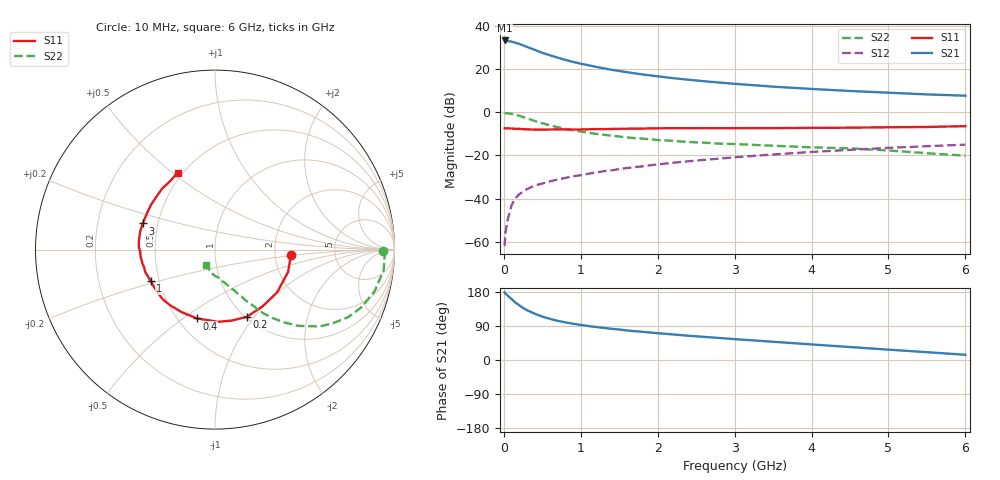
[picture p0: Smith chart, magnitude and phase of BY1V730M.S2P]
! SIEMENS Small Signal Semiconductors
! BFY420
! Si NPN RF SIEGET Grounded Emitter Transistor in MICRO-X
! VCE = 1.75 V  IC = 30 mA
! Common Emitter S-Parameters:  October  1996
# GHz  S  MA  R  50
!  f  S11  S21  S12  S22
! GHz  MAG  ANG  MAG  ANG  MAG  ANG  MAG  ANG
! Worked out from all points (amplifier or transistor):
!   36 points, 10 MHz to 6 GHz, reference 50 ohm
!   highest |S21| = 33.2 dB at 10 MHz (marker M1)
!   |S21| within 3 dB of that: start of sweep to 302.7 MHz
!   unconditionally stable (mu >= 1): start of sweep to 12.17 MHz; 1.57 GHz to end of sweep
!   at 250 MHz: K = 0.37, MSG = 33.8 dB, |S12| = -36.8 dB
!   at 1.4 GHz: K = 0.98, MSG = 23.3 dB, |S12| = -26.9 dB
!   at 6 GHz: K = 1.07, MAG = 9.7 dB, |S12| = -15.0 dB
!   S11 on the Smith chart (normalised r, x): 10 MHz: 2.47, -0.19; 200 MHz: 1.02, -0.92; 400 MHz: 0.62, -0.56; 1 GHz: 0.45, -0.19; 3 GHz: 0.41, +0.15; 6 GHz: 0.47, +0.52
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0.01  0.4257 -4.2  45.69 178.5  0.0008 117.0  0.9381 -0.4
0.02  0.4227 -7.6  45.66 175.3  0.0016 75.3  0.9451 -2.0
0.1  0.4201 -34.6  42.92 161.0  0.007 81.0  0.9198 -14.5
0.15  0.4126 -49.6  40.46 151.5  0.0102 72.7  0.8784 -21.3
0.2  0.4143 -64.5  38.05 144.5  0.0127 70.4  0.8311 -27.0
0.25  0.4064 -76.5  35.16 137.2  0.0145 67.0  0.7739 -32.0
0.3  0.4027 -87.6  32.48 131.5  0.0167 65.6  0.7245 -36.2
0.4  0.3965 -104.8  27.78 122.3  0.0201 61.9  0.6303 -42.4
0.5  0.3948 -118.1  23.69 114.4  0.0225 60.5  0.5564 -46.7
0.6  0.3985 -128.9  20.72 108.6  0.0252 60.2  0.4981 -49.9
0.7  0.4018 -136.5  18.29 103.4  0.0279 60.7  0.4513 -52.5
0.8  0.3996 -143.6  16.22 99.2  0.0303 59.7  0.4123 -54.4
1  0.3991 -154.1  13.25 92.5  0.0349 60.5  0.358 -57.0
1.1  0.4034 -159.1  12.19 89.6  0.0379 60.2  0.3359 -58.6
1.4  0.4114 -168.9  9.577 82.4  0.0453 61.1  0.2883 -61.7
1.6  0.4162 -174.6  8.411 78.0  0.0512 60.5  0.2621 -63.8
2.2  0.427 173.1  6.135 67.4  0.0679 58.2  0.2178 -69.5
3  0.4283 160.1  4.541 55.1  0.0908 53.4  0.1839 -76.2
3.5  0.4296 152.0  3.908 48.1  0.1053 49.7  0.168 -80.8
4.5  0.4394 138.2  3.101 34.2  0.1348 41.0  0.1462 -90.1
5.5  0.4566 123.0  2.586 20.6  0.1642 31.2  0.1128 -108.0
6  0.4767 115.9  2.414 13.8  0.178 26.4  0.099 -121.8
